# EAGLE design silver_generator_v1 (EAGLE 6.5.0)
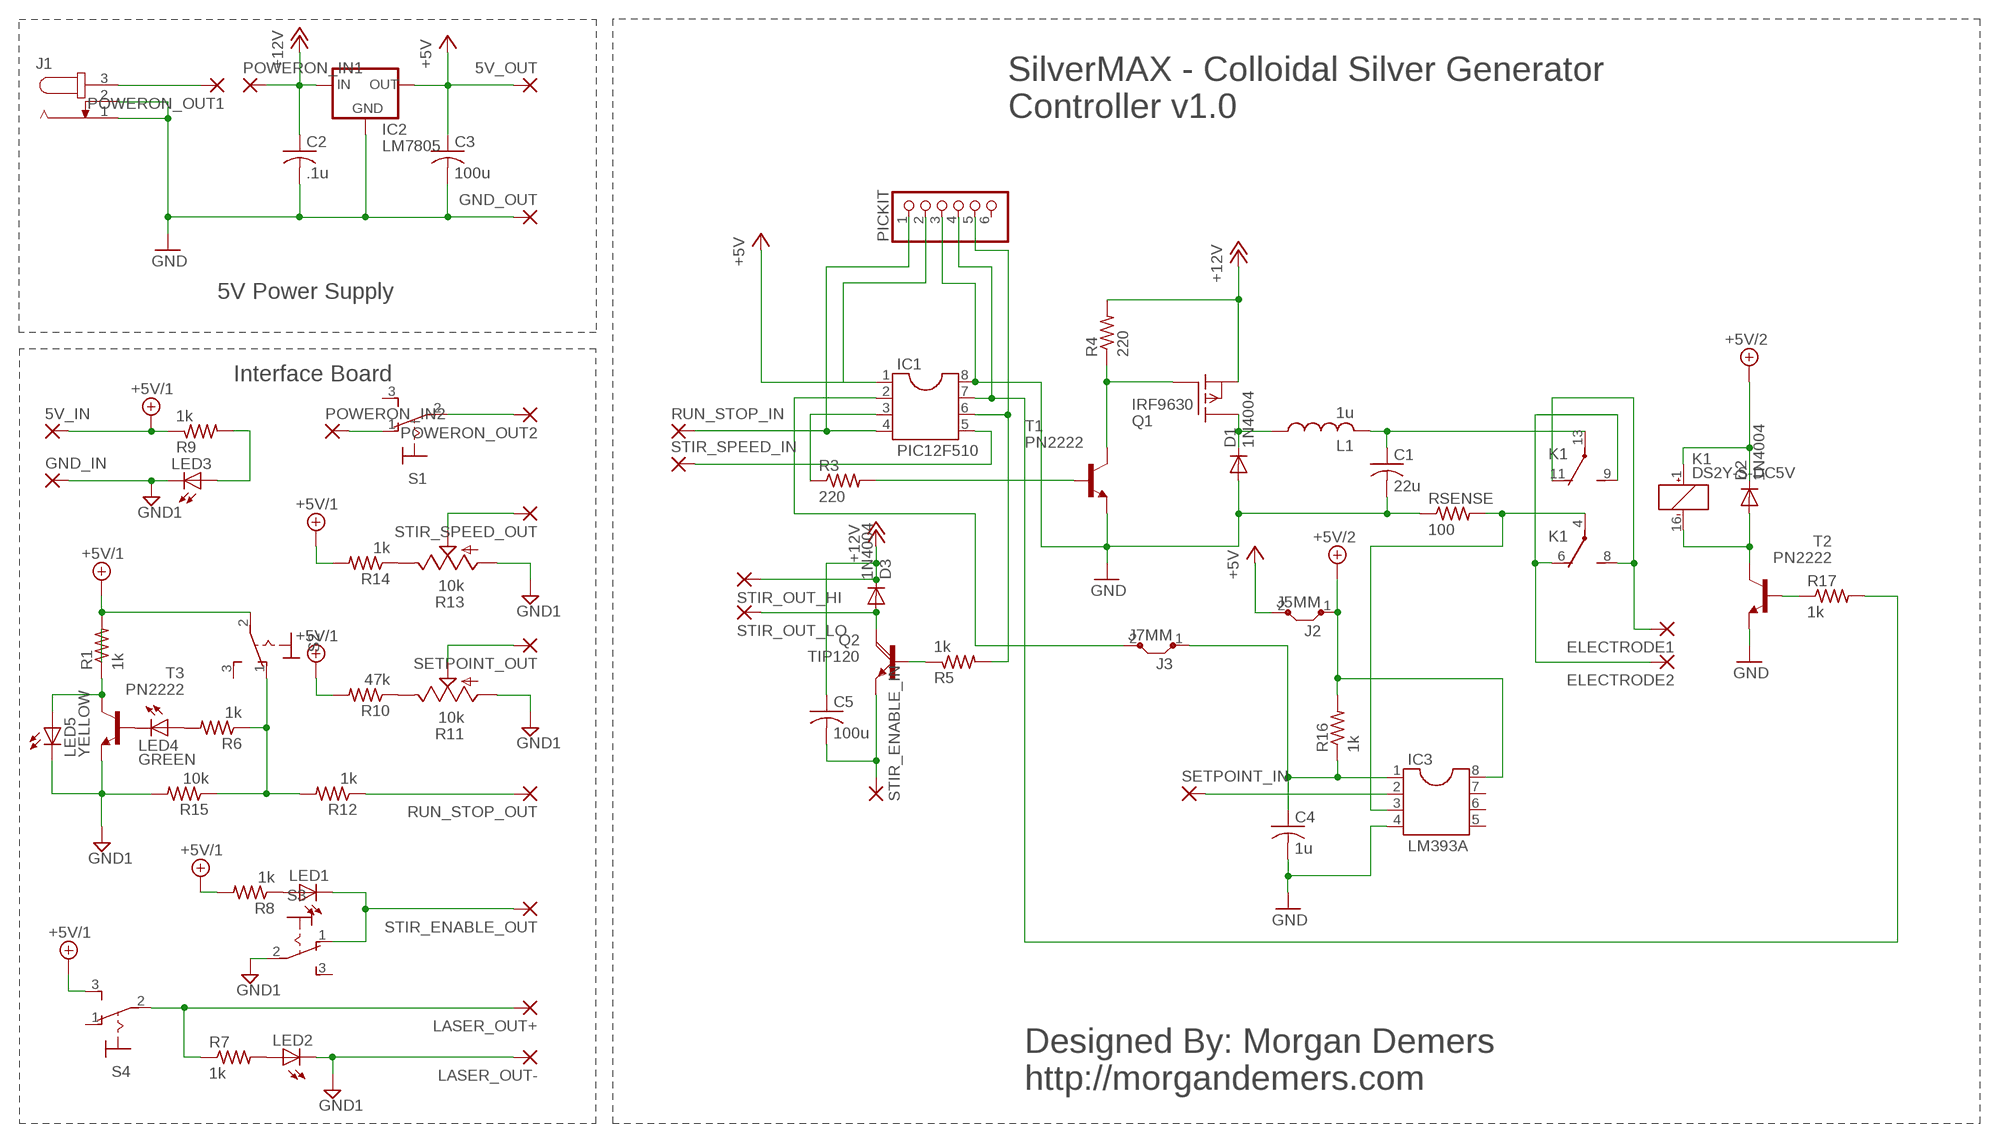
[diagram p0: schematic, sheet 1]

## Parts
5V_IN  1,6/0,9  [1,6/0,9]
5V_OUT  1,6/0,9  [1,6/0,9]
C1  22u  C-US025-050X050  [C025-050X050]
C2  .1u  C-US025-025X050  [C025-025X050]
C3  100u  C-US025-050X050  [C025-050X050]
C4  1u  C-US025-050X050  [C025-050X050]
C5  100u  C-US050-075X075  [C050-075X075]
D1  1N4004  [DO41-10]
D2  1N4004  [DO41-10]
D3  1N4004  [DO41-10]
ELECTRODE1  1,6/0,9  [1,6/0,9]
ELECTRODE2  1,6/0,9  [1,6/0,9]
GND_IN  1,6/0,9  [1,6/0,9]
GND_OUT  1,6/0,9  [1,6/0,9]
IC1  PIC12F510  DIL8S  [SOCKET-08]
IC2  LM7805  78XXL  [78XXL]
IC3  LM393A  DIL8S  [SOCKET-08]
J1  JACK-PLUG1  [SPC4078]
J2  J5MM  [05]
J3  J7MM  [07]
K1  DS2Y-S-DC5V  [DS2Y]
L1  1u  L-US0204/5  [0204/5]
LASER_OUT+  1,6/0,9  [1,6/0,9]
LASER_OUT-  1,6/0,9  [1,6/0,9]
LED1  LED3MM  [LED3MM]
LED2  LED3MM  [LED3MM]
LED3  LED3MM  [LED3MM]
LED4  GREEN  LED3MM  [LED3MM]
LED5  YELLOW  LED3MM  [LED3MM]
PICKIT  PINHD-1X6  [1X06]
POWERON_IN1  1,6/0,9  [1,6/0,9]
POWERON_IN2  1,6/0,9  [1,6/0,9]
POWERON_OUT1  1,6/0,9  [1,6/0,9]
POWERON_OUT2  1,6/0,9  [1,6/0,9]
Q1  IRF9630  IRF9530  [TO220]
Q2  TIP120  [TO220AH]
R1  1k  R-US_0204/5  [0204/5]
R3  220  R-US_0204/7  [0204/7]
R4  220  R-US_0204/5  [0204/5]
R5  1k  R-US_0207/12  [0207/12]
R6  1k  R-US_0204/5  [0204/5]
R7  1k  R-US_0204/5  [0204/5]
R8  1k  R-US_0204/5  [0204/5]
R9  1k  R-US_0204/5  [0204/5]
R10  47k  R-US_0204/5  [0204/5]
R11  10k  TRIM_US-B25P  [B25P]
R12  1k  R-US_0204/5  [0204/5]
R13  10k  TRIM_US-B25P  [B25P]
R14  1k  R-US_0204/5  [0204/5]
R15  10k  R-US_0204/5  [0204/5]
R16  1k  R-US_0204/5  [0204/5]
R17  1k  R-US_0204/7  [0204/7]
RSENSE  100  R-US_0204/5  [0204/5]
RUN_STOP_IN  1,6/0,9  [1,6/0,9]
RUN_STOP_OUT  1,6/0,9  [1,6/0,9]
S1  M9040P  [M9040P]
S2  M9040P  [M9040P]
S3  M9040P  [M9040P]
S4  M9040P  [M9040P]
SETPOINT_IN  1,6/0,9  [1,6/0,9]
SETPOINT_OUT  1,6/0,9  [1,6/0,9]
STIR_ENABLE_IN  1,6/0,9  [1,6/0,9]
STIR_ENABLE_OUT  1,6/0,9  [1,6/0,9]
STIR_OUT_HI  1,6/0,9  [1,6/0,9]
STIR_OUT_LO  1,6/0,9  [1,6/0,9]
STIR_SPEED_IN  1,6/0,9  [1,6/0,9]
STIR_SPEED_OUT  1,6/0,9  [1,6/0,9]
T1  PN2222  -NPN-TO92-EBC  [TO92-EBC]
T2  PN2222  -NPN-TO92-EBC  [TO92-EBC]
T3  PN2222  -NPN-TO92-EBC  [TO92-EBC]

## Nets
+5V: 5V_OUT.1(P) C3.1 IC1.1 IC2.OUT J2.2 PICKIT.2
+5V/1: 5V_IN.1(P) R1.2 R8.2 R9.1 R10.2 R14.2 S2.2(P) S4.3(S)
+5V/2: D2.C IC3.8 J2.1 K1.1(1:+) R16.2
+12V: C2.1 C5.1 D3.C IC2.IN POWERON_IN1.1(P) Q1.3(S) R4.2 STIR_OUT_HI.1(P)
GND: C1.2 C2.2 C3.2 C4.2 D1.A GND_OUT.1(P) IC1.8 IC2.GND IC3.4 J1.1 J1.2 PICKIT.3 RSENSE.1 T1.E T2.E
GND1: GND_IN.1(P) LASER_OUT-.1(P) LED2.K(C) LED3.K(C) LED5.K(C) R11.A R13.A R15.2 S3.2(P) T3.E
N$1: IC1.3 R3.1
N$2: R3.2 T1.B
N$3: LED1.K(C) S3.1(O) STIR_ENABLE_OUT.1(P)
N$4: IC3.2 SETPOINT_IN.1(P)
N$5: Q1.1(G) R4.1 T1.C
N$6: D3.A Q2.C STIR_OUT_LO.1(P)
N$7: C1.1 K1.13(3:P) L1.2
N$8: IC1.6 PICKIT.5 R5.2
N$9: IC1.4 PICKIT.1 RUN_STOP_IN.1(P)
N$10: D1.C L1.1 Q1.2(D)
N$11: POWERON_IN2.1(P) S1.1(O)
N$12: IC3.3 K1.4(2:P) RSENSE.2
N$13: R6.1 R12.2 R15.1 S2.1(O)
N$14: LED2.A R7.2
N$15: ELECTRODE2.1(P) K1.6(2:O) K1.9(3:S)
N$16: LED1.A R8.1
N$17: R13.S STIR_SPEED_OUT.1(P)
N$18: LED3.A R9.2
N$19: IC1.7 PICKIT.4 R17.2
N$20: R10.1 R11.E
N$21: ELECTRODE1.1(P) K1.8(2:S) K1.11(3:O)
N$22: IC1.2 J3.2
N$24: LED5.A R1.1 T3.C
N$25: LED4.K(C) T3.B
N$26: LED4.A R6.2
N$27: LASER_OUT+.1(P) R7.1 S4.2(P)
N$28: C5.2 Q2.E STIR_ENABLE_IN.1(P)
N$29: IC1.5 STIR_SPEED_IN.1(P)
N$30: R13.E R14.1
N$31: Q2.B R5.1
N$32: R12.1 RUN_STOP_OUT.1(P)
N$33: R11.S SETPOINT_OUT.1(P)
N$34: R17.1 T2.B
N$35: D2.A K1.16(1:-) T2.C
N$36: J1.3 POWERON_OUT1.1(P)
N$39: POWERON_OUT2.1(P) S1.2(P)
N$40: C4.1 IC3.1 J3.1 R16.1
Unconnected: IC3.5 IC3.6 IC3.7 PICKIT.6 S1.3(S) S2.3(S) S3.3(S) S4.1(O)

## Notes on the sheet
- SilverMAX - Colloidal Silver Generator
  Controller v1.0
- 5V Power Supply
- Interface Board
- Designed By: Morgan Demers
  http://morgandemers.com

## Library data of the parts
5V_IN 5V_OUT ELECTRODE1 ELECTRODE2 GND_IN GND_OUT LASER_OUT+ LASER_OUT- POWERON_IN1 POWERON_IN2 POWERON_OUT1 POWERON_OUT2 RUN_STOP_IN RUN_STOP_OUT SETPOINT_IN SETPOINT_OUT STIR_ENABLE_IN STIR_ENABLE_OUT STIR_OUT_HI STIR_OUT_LO STIR_SPEED_IN STIR_SPEED_OUT = wirepad:1,6/0,9: THROUGH-HOLE PAD
C1-C5 = resistor:C-US: CAPACITOR, American symbol
D1-D3 = diode:1N4004: DIODE
IC1 IC3 = ic-package:DIL8: Dual In Line / Socket
IC2 = v-reg:78XXL: VOLTAGE REGULATOR
J1 = con-jack:JACK-PLUG: DC POWER JACK Power Jack, DC, Right Angle, Through Hole, Rated 5A at 16VDC, PC Terminals Distributor: Farnell (www.Farnell.de) Drawing: 84N1161.pdf / 84N1162.pdf Manufacturer: SPC Technology (www.spctechnology.com) Type: SPC4077 / SPC 4078; OC_FARNELL: unknown; OC_NEWARK: unknown
J2 J3 = jumper:J: Bridge
K1 = relay:DS2Y-S-DC*: MINIATURE RELAY NAiS Source: http://www.mew-europe.com/.. en_ds_61005_0023.pdf; MPN: DS2Y-S-DC5V; OC_FARNELL: unknown; OC_NEWARK: 13P3268
L1 = resistor:L-US: INDUCTOR, American symbol
LED1-LED5 = led:LED: LED
PICKIT = pinhead:PINHD-1X6: PIN HEADER
Q1 = transistor-fet:IRF9530: P-Channel Enhancement MOSFET (HEXFET); -100V; -12A; 0,3Ohm
Q2 = transistor-power:TIP120: NPN DARLINGTON TRANSISTOR
R1 R3-R10 R12 R14-R17 RSENSE = resistor:R-US_: RESISTOR, American symbol
R11 R13 = pot:TRIM_US-: POTENTIOMETER
S1-S4 = switch:M9040P: TOGGLE SWITCH Marquardt
T1-T3 = transistor:*-NPN-: NPN Transistror BF959 corrected 2008.03.06

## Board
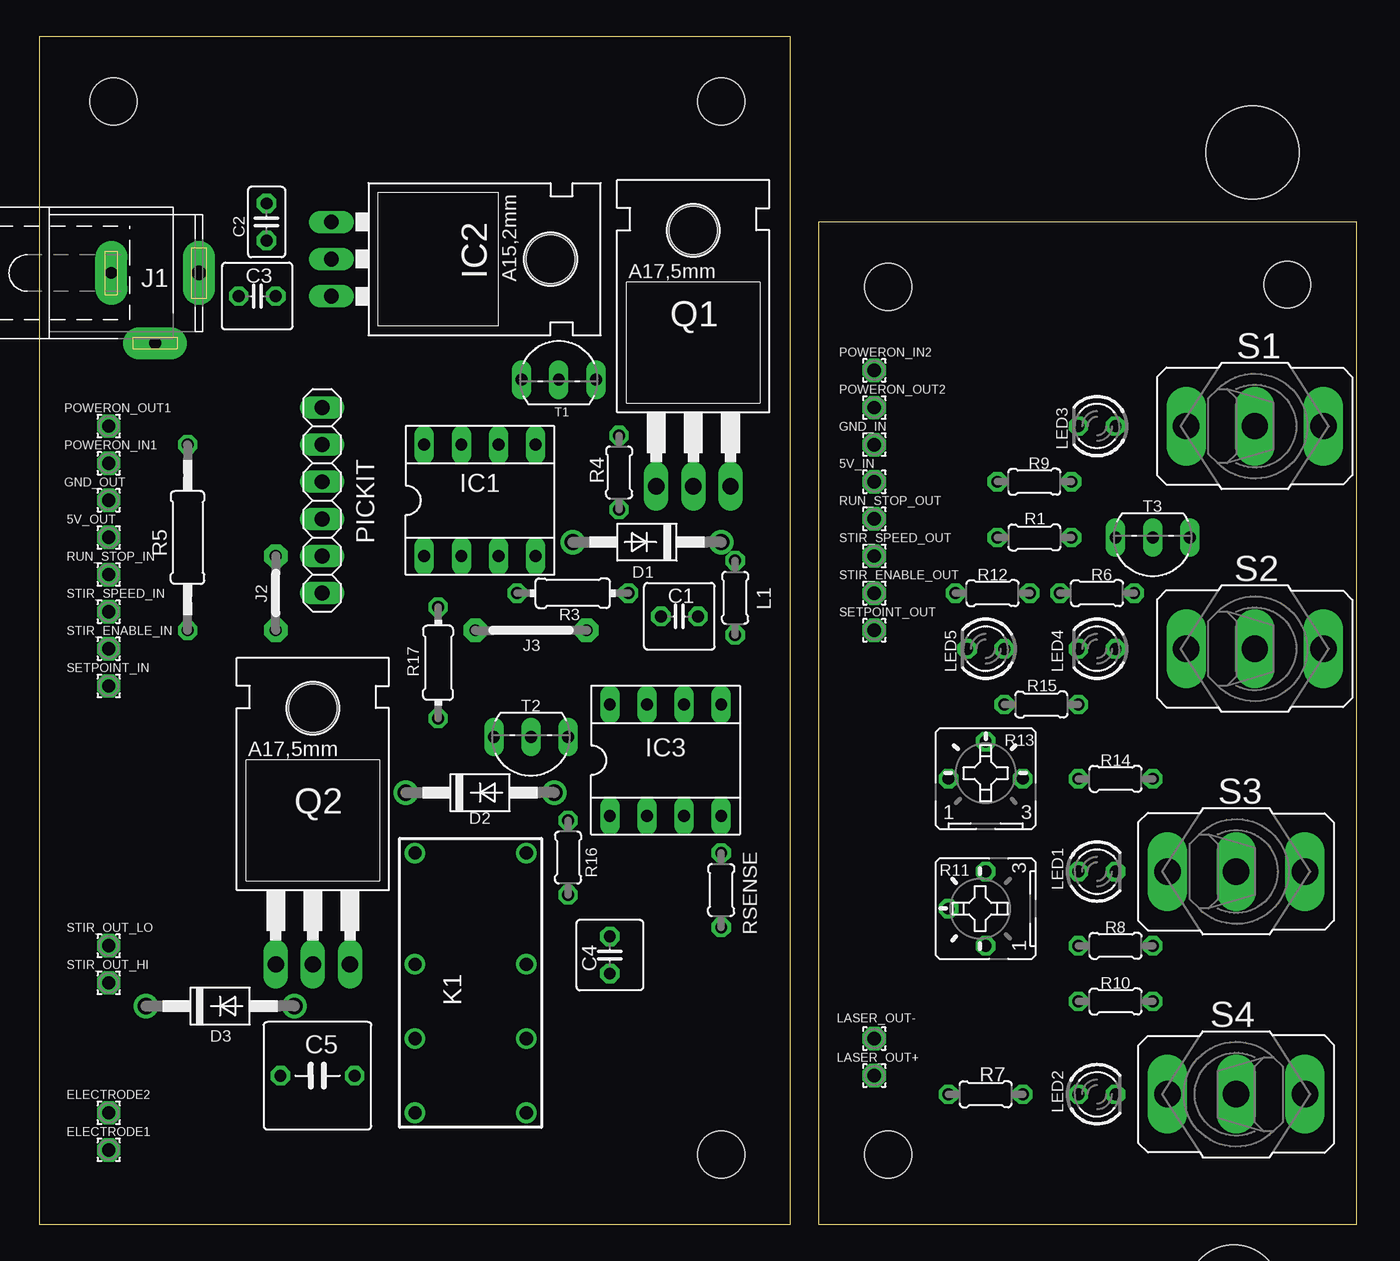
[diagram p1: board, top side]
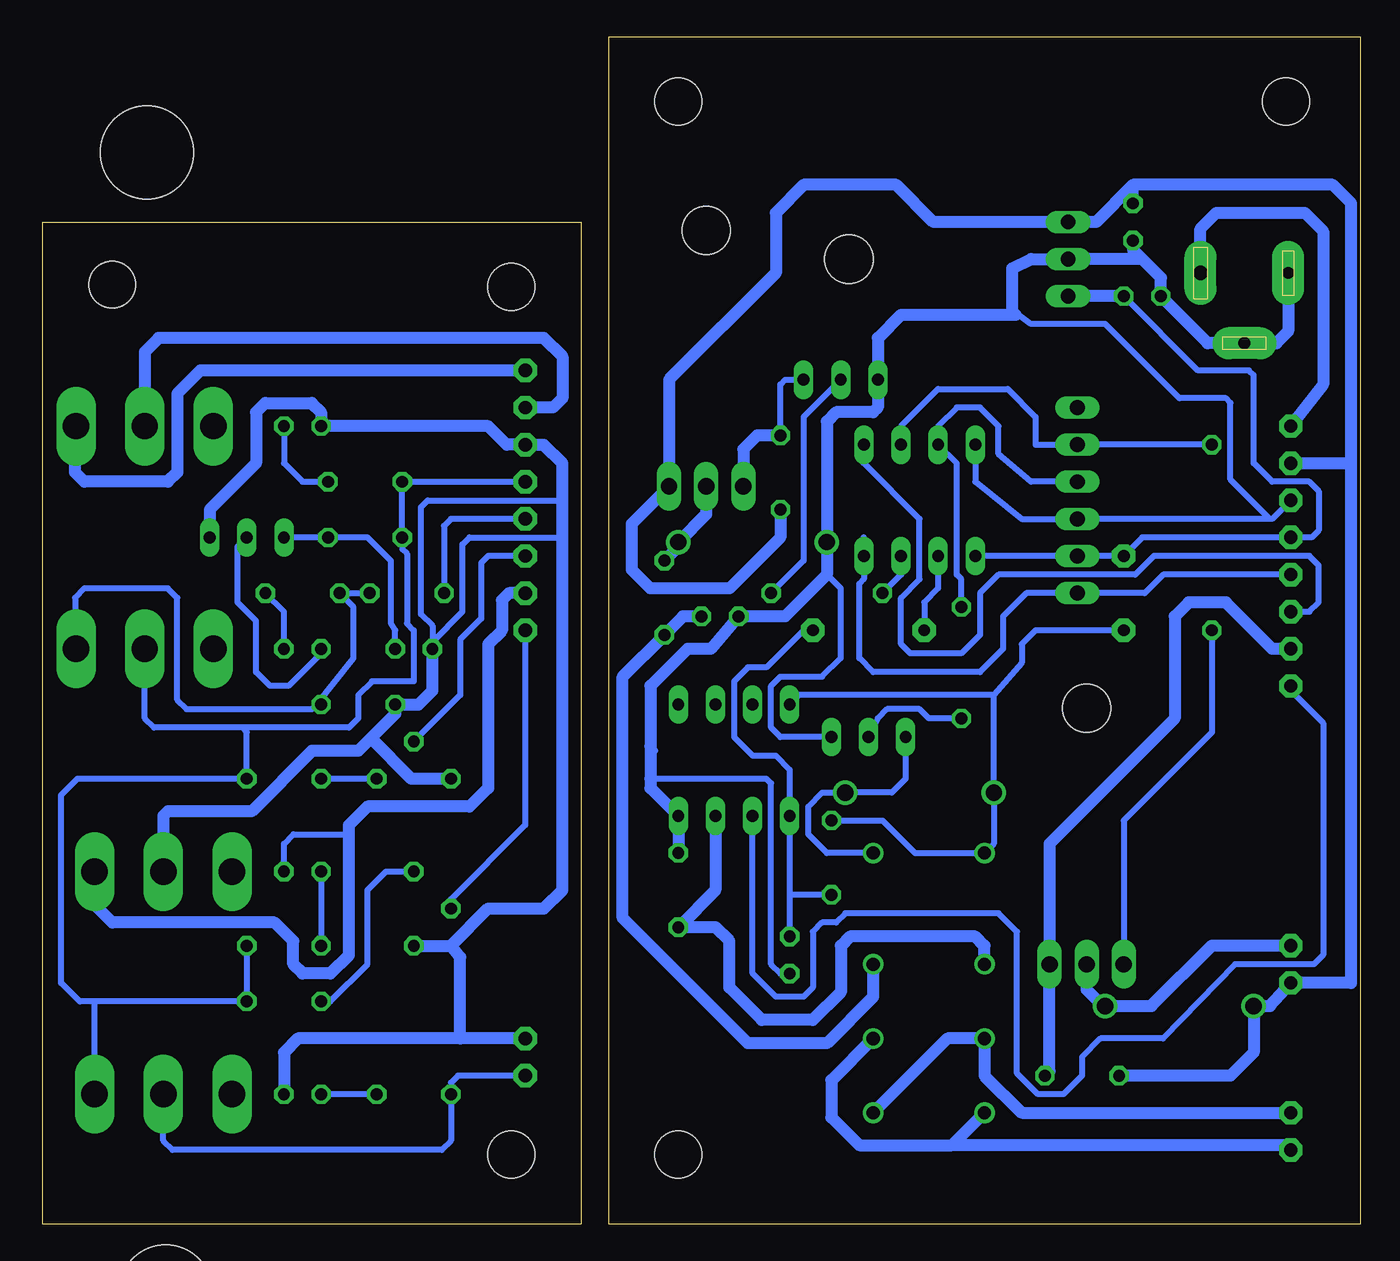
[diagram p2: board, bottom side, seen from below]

Size 90.17 x 81.27 mm. Coordinates in mm from the lower left corner, seen from the top.
Outline: 0,0 51.42,0 51.42,81.27 0,81.27 0,0
Outline: 53.34,68.58 53.34,0 90.17,0 90.17,68.58 53.34,68.58
Copper layers (1*16): Top 0.035mm / dielectric 1.5mm / Bottom 0.035mm
Design rules "default": minimum track width 10mil, minimum drill 24mil, track to track 8mil, track to pad 8mil, pad to pad 8mil, via to via 8mil, smd to smd 8mil, copper to edge 40mil, drill to drill 8mil, minimum pad ring 10mil, minimum via ring 8mil, stop-mask expansion 4mil, vias tented up to drill 0mil, thermal gap 10mil
Holes 3.2 mm at 5.08,76.83 46.67,76.83 46.67,4.76 58.1,4.76 85.41,64.29 58.1,64.14
Holes 6.35 mm at 83.03,73.34 81.76,-4.6

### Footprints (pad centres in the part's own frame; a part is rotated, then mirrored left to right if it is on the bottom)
1,6/0,9 = drill 0.914 pad 1.6 octagon: 1 0,0
C025-050X050 = drill 0.813 octagon: 1 -1.27,0; 2 1.27,0
C025-025X050 = drill 0.813 octagon: 1 -1.27,0; 2 1.27,0
C050-075X075 = drill 0.813 octagon: 1 -2.54,0; 2 2.54,0
DO41-10 = drill 1.118: A 5.08,0; C -5.08,0
SOCKET-08 = drill 0.813 long: 1 -3.81,-3.81; 2 -1.27,-3.81; 3 1.27,-3.81; 4 3.81,-3.81; 5 3.81,3.81; 6 1.27,3.81; 7 -1.27,3.81; 8 -3.81,3.81
78XXL = drill 1.016 long: GND 0,-3.81; IN -2.54,-3.81; OUT 2.54,-3.81 | hole 3.302: 0,11.176
SPC4078 = drill 0.8 pad 2.184 long: 1 -3,0; 2 0,-4.8 | drill 1 pad 2.184 long: 3 3,0
05 = drill 0.813 pad 1.6 octagon: 1 -2.54,0; 2 2.54,0
07 = drill 0.813 pad 1.6 octagon: 1 -3.81,0; 2 3.81,0
DS2Y = drill 0.9: 1 -8.89,-3.81; 4 -1.27,-3.81; 6 3.81,-3.81; 8 8.89,-3.81; 9 8.89,3.81; 11 3.81,3.81; 13 -1.27,3.81; 16 -8.89,3.81
0204/5 = drill 0.813 octagon: 1 -2.54,0; 2 2.54,0
LED3MM = drill 0.813 octagon: A -1.27,0; K 1.27,0
1X06 = drill 1.016 long: 1 -6.35,0; 2 -3.81,0; 3 -1.27,0; 4 1.27,0; 5 3.81,0; 6 6.35,0
TO220 = drill 1.118 long: 1 -2.54,-6.35; 2 0,-6.35; 3 2.54,-6.35 | hole 3.302: 0,11.176
TO220AH = drill 1.118 long: B -2.54,-6.35; C 0,-6.35; E 2.54,-6.35 | hole 3.302: 0,11.176
0204/7 = drill 0.813 octagon: 1 -3.81,0; 2 3.81,0
0207/12 = drill 0.813 octagon: 1 -6.35,0; 2 6.35,0
B25P = drill 0.813 octagon: A -2.54,0; E 2.54,0; S 0,2.54
M9040P = drill 1.803 long: 1 0,4.699; 2 0,0; 3 0,-4.699
TO92-EBC = drill 0.813 long: B 0,-1.27; C 2.54,-1.27; E -2.54,-1.27

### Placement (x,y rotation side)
5V_IN  57.15,50.8 0 top
5V_OUT  4.76,46.99 0 top
C1  43.81,41.59 180 top
C2  15.56,68.58 270 top
C3  14.92,63.5 180 top
C4  39.05,18.41 270 top
C5  19.05,10.16 0 top
D1  41.59,46.67 180 top
D2  30.16,29.53 0 top
D3  12.38,14.92 0 top
ELECTRODE1  4.76,5.08 0 top
ELECTRODE2  4.76,7.62 0 top
GND_IN  57.15,53.34 0 top
GND_OUT  4.76,49.53 0 top
IC1  30.16,49.53 0 top
IC2  23.81,66.04 270 top
IC3  42.86,31.75 0 top
J1  7.94,65.09 0 top
J2  16.19,43.18 90 top
J3  33.66,40.64 180 top
K1  29.53,16.51 270 top
L1  47.62,42.86 270 top
LASER_OUT+  57.15,10.16 0 top
LASER_OUT-  57.15,12.7 0 top
LED1  72.39,24.13 0 top
LED2  72.39,8.89 0 top
LED3  72.39,54.61 180 top
LED4  72.39,39.37 180 top
LED5  64.77,39.37 180 top
PICKIT  19.37,49.53 90 top
POWERON_IN1  4.76,52.07 0 top
POWERON_IN2  57.15,58.42 0 top
POWERON_OUT1  4.76,54.61 0 top
POWERON_OUT2  57.15,55.88 0 top
Q1  44.77,56.83 0 top
Q2  18.73,24.13 0 top
R1  68.1,46.99 180 top
R3  36.51,43.18 0 top
R4  39.69,51.44 270 top
R5  10.16,46.99 90 top
R6  72.39,43.18 0 top
R7  64.77,8.89 0 top
R8  73.66,19.05 0 top
R9  68.1,50.8 0 top
R10  73.66,15.24 0 top
R11  64.77,21.59 90 top
R12  65.25,43.18 0 top
R13  64.77,30.48 0 top
R14  73.66,30.48 0 top
R15  68.58,35.56 180 top
R16  36.2,25.08 90 top
R17  27.3,38.42 90 top
RSENSE  46.67,22.86 270 top
RUN_STOP_IN  4.76,44.45 0 top
RUN_STOP_OUT  57.15,48.26 0 top
S1  83.19,54.61 270 top
S2  83.19,39.37 270 top
S3  81.92,24.13 270 top
S4  81.92,8.89 90 top
SETPOINT_IN  4.76,36.83 0 top
SETPOINT_OUT  57.15,40.64 0 top
STIR_ENABLE_IN  4.76,39.37 0 top
STIR_ENABLE_OUT  57.15,43.18 0 top
STIR_OUT_HI  4.76,16.51 0 top
STIR_OUT_LO  4.76,19.05 0 top
STIR_SPEED_IN  4.76,41.91 0 top
STIR_SPEED_OUT  57.15,45.72 0 top
T1  35.56,59.05 0 top
T2  33.66,32.07 180 top
T3  76.2,45.72 180 top

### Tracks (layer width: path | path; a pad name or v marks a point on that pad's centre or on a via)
+5V
  Bottom 0.406: IC1.1 PICKIT.2 J2.2 14.92,46.99 5V_OUT.1 3.33,46.99 2.86,47.47 2.86,50.16 3.49,50.8 6.03,50.8 7.3,52.07 7.3,58.1 7.62,58.42 11.11,58.42 C3.1
  Bottom 0.813: C3.1 IC2.OUT
+5V/1
  Bottom 0.406: 5V_IN.1 R9.1 R1.2 65.56,46.2 65.25,45.88 65.25,41.12 64.77,40.64 64.77,37.15 67.63,37.15 68.58,36.2 68.58,34.61 69.22,33.97 76.52,33.97 | 76.52,33.97 82.55,33.97 83.19,34.61 S2.2 | R10.2 76.83,15.24 | 76.83,15.24 86.68,15.24 | R8.2 76.2,15.88 76.83,15.24 | 76.52,33.97 76.2,33.66 R14.2 87.79,30.48 88.9,29.37 88.9,16.51 87.63,15.24 86.68,15.24 | S4.3 86.61,15.18 86.68,15.24
+5V/2
  Bottom 0.406: 25.08,36.2 23.18,38.42 23.18,39.69 22.23,40.64 J2.1 | 25.08,36.2 38.42,36.2 IC3.8 | 25.08,36.2 D2.C 25.08,26.04 K1.1 30.48,25.4 32.7,27.62 R16.2
+12V
  Bottom 0.813: 15.56,71.12 1.91,71.12 0.64,69.85 0.64,52.07 | 15.56,71.12 18.1,68.58 IC2.IN 29.21,68.58 31.75,71.12 38.1,71.12 40.01,69.22 40.01,65.09 47.31,57.78 Q1.3 49.85,47.94 49.85,44.77 48.58,43.5 43.18,43.5 39.69,46.99 R4.2 | C2.1 15.56,71.12 | 0.64,52.07 0.64,16.51 STIR_OUT_HI.1 6.19,14.92 D3.C 7.3,11.75 8.89,10.16 C5.1 | POWERON_IN1.1 0.64,52.07
GND
  Bottom 0.406: IC1.8 26.35,50.8 23.18,48.26 PICKIT.3 | GND_OUT.1 6.03,48.26 6.19,48.26 | 6.19,48.26 PICKIT.3 | PICKIT.3 18.73,48.26 | 23.51,62.32 22.54,61.59 17.46,61.59 12.38,56.52 9.21,56.52 8.89,56.2 8.89,50.96 6.19,48.26 | 23.51,62.32 23.81,62.55 | 23.6,62.23 23.51,62.32 | C4.2 39.69,17.14 40.32,17.78 40.32,30.16 40.64,30.48 48.58,30.48 | 48.26,32.38 48.58,32.7 | T2.E 39.69,33.34 40.32,33.97 40.32,36.83 39.69,37.47 36.83,37.47 35.56,38.73 35.56,43.5 36.51,44.45
  Bottom 0.813: 14.92,66.04 13.65,64.77 C3.2 10.44,60.29 J1.2 5.75,60.29 4.94,61.1 J1.1 | 14.92,66.04 IC2.GND 22.54,66.04 23.81,65.41 23.81,62.55 | C2.2 15.56,66.67 14.92,66.04 | 23.6,62.23 31.43,62.23 33.02,60.64 T1.E 33.02,55.88 33.34,55.56 35.88,55.56 36.51,54.93 D1.A 36.51,44.45 39.37,41.59 C1.2 44.45,39.37 46.04,39.37 48.58,36.83 48.58,32.7 48.58,30.48 48.58,29.84 IC3.4 RSENSE.1
GND1
  Bottom 0.406: 54.61,49.53 63.82,49.53 64.29,49.05 64.29,41.75 63.5,40.96 63.5,39.85 | 63.5,39.85 61.44,41.91 61.44,46.51 60.96,46.99 54.93,46.99 54.77,46.83 | 63.5,39.85 LED5.K
  Bottom 0.813: R11.A 62.23,19.05 | 62.23,19.05 61.59,18.26 61.59,12.7 | 62.23,19.05 59.69,21.59 55.88,21.59 54.61,22.86 54.61,49.53 54.61,52.07 55.88,53.34 GND_IN.1 58.42,53.34 59.69,54.61 LED3.K 71.12,55.56 71.75,56.2 74.93,56.2 75.56,55.56 75.56,52.07 78.74,48.9 T3.E | LASER_OUT-.1 61.59,12.7 | 61.59,12.7 72.71,12.7 73.66,11.75 LED2.K | 67.71,33.26 66.04,34.92 R15.2 64.45,35.56 63.5,36.51 LED5.K | 67.71,33.26 68.58,32.38 71.75,32.38 75.88,28.26 81.6,28.26 81.92,27.94 S3.2 | R13.A 64.93,30.48 67.71,33.26
N$1
  Bottom 0.406: IC1.3 31.43,44.45 R3.1
N$2
  Bottom 0.406: R3.2 38.1,45.4 38.1,55.24 T1.B
N$3
  Bottom 0.406: LED1.K 73.66,26.04 73.03,26.67 69.22,26.67
  Bottom 0.813: S3.1 86.68,24.07 86.68,21.91 85.41,20.64 74.3,20.64 73.03,19.37 73.03,17.78 72.39,17.14 70.48,17.14 69.22,18.41 69.22,26.67 69.22,27.3 67.94,28.57 60.96,28.57 59.69,29.84 59.69,39.69 58.74,40.64 58.74,42.7 58.26,43.18 STIR_ENABLE_OUT.1
N$4
  Bottom 0.406: IC3.2 41.59,17.14 40.01,15.56 38.1,15.56 37.47,16.19 37.47,20 36.83,20.64 35.88,20.64 35.24,21.27 24.77,21.27 23.5,20 23.5,10.32 22.07,8.89 20.32,8.89 19.05,10.16 19.05,11.43 17.78,12.7 13.49,12.7 8.57,17.78 3.17,17.78 2.54,18.41 2.54,34.29 4.76,36.51 SETPOINT_IN.1
N$5
  Bottom 0.406: R4.1 39.69,57.47 39.37,57.78 T1.C
  Bottom 0.813: R4.1 41.27,53.98 42.23,53.02 Q1.1
N$6
  Bottom 0.813: STIR_OUT_LO.1 10.16,19.05 14.29,14.92 D3.A 17.62,14.92 18.73,16.03 Q2.C
N$7
  Bottom 0.813: C1.1 46.35,41.59 L1.2 50.48,37.47 50.48,20.95 41.91,12.38 36.51,12.38 33.34,15.56 K1.13
N$8
  Bottom 0.406: IC1.6 31.43,54.61 28.89,57.15 24.13,57.15 22.23,55.24 22.23,53.34 PICKIT.5 | 19.68,53.66 PICKIT.5 | R5.2 PICKIT.5
N$9
  Bottom 0.406: 33.97,46.99 IC1.4 33.97,44.13 34.29,43.81 34.29,38.73 33.34,37.78 26.04,37.78 24.45,39.37 24.45,41.59 22.86,43.18 PICKIT.1 14.76,43.18 13.49,44.45 RUN_STOP_IN.1
N$10
  Bottom 0.813: L1.1 46.67,46.35 D1.C 44.77,48.58 Q1.2
N$11
  Bottom 0.813: POWERON_IN2.1 79.38,58.42 80.96,56.83 80.96,51.44 81.6,50.8 87.31,50.8 87.95,51.44 87.95,54.55 S1.1
N$12
  Bottom 0.813: IC3.3 44.13,22.86 RSENSE.2 44.13,20.32 43.18,19.37 43.18,16.19 40.96,13.97 37.47,13.97 35.56,15.88 35.56,19.05 34.92,19.68 26.35,19.68 25.72,19.05 K1.4
N$13
  Bottom 0.406: 71.44,35.56 68.9,38.73 68.9,42.23 R6.1 R12.2 | R15.1 71.44,35.56 | 71.44,35.56 71.75,35.24 80.33,35.24 80.96,35.88 80.96,42.86 81.6,43.5 87.31,43.5 87.95,42.86 87.95,39.43 S2.1
N$14
  Bottom 0.406: R7.2 LED2.A
N$15
  Bottom 0.813: K1.9 28.26,12.7 K1.6 25.72,10.16 23.18,7.62 ELECTRODE2.1
N$16
  Bottom 0.406: LED1.A R8.1
N$17
  Bottom 0.406: STIR_SPEED_OUT.1 59.69,45.72 60.17,45.24 60.17,41.43 61.59,40.01 61.59,36.2 R13.S
N$18
  Bottom 0.406: LED3.A 73.66,52.07 72.39,50.8 R9.2
N$19
  Bottom 0.406: PICKIT.4 22.54,50.8 24.77,52.7 24.77,54.61 26.04,55.88 27.62,55.88 28.89,54.61 IC1.7 27.62,52.07 27.62,44.45 27.3,44.13 R17.2
N$20
  Bottom 0.406: R10.1 70.48,15.24 67.94,17.78 67.94,22.86 66.67,24.13 R11.E
N$21
  Bottom 0.813: K1.11 36.2,9.84 36.2,7.3 34.29,5.4 27.94,5.4 | K1.8 27.94,5.4 | ELECTRODE1.1 5.08,5.4 27.94,5.4
N$22
  Bottom 0.406: IC1.2 28.89,43.5 29.84,42.55 J3.2
N$24
  Bottom 0.406: LED5.A 66.04,40.64 66.36,41.12 66.36,45.4 67.94,46.99 R1.1 T3.C
N$25
  Bottom 0.406: LED4.K 71.12,39.05 73.34,36.83 74.61,36.83 75.56,37.78 75.56,41.27 76.83,42.55 76.83,46.35 T3.B
N$26
  Bottom 0.406: LED4.A 73.66,41.91 R6.2
N$27
  Bottom 0.406: LASER_OUT+.1 61.75,10.16 62.23,9.68 R7.1 62.23,5.71 62.87,5.08 81.28,5.08 81.92,5.71 S4.2
N$28
  Bottom 0.813: STIR_ENABLE_IN.1 6.03,39.37 9.21,42.55 11.75,42.55 12.7,41.59 12.7,34.61 21.27,26.04 Q2.E 21.27,10.48 C5.2
N$29
  Bottom 0.406: STIR_SPEED_IN.1 3.49,41.91 2.86,42.55 2.86,45.09 3.49,45.72 14.13,45.72 15.4,44.45 24.77,44.45 26.04,43.18 26.04,40.32 27.3,39.05 30.8,39.05 31.43,39.69 31.43,42.86 30.16,44.13 30.16,48.26 33.97,52.07 IC1.5
N$30
  Bottom 0.406: R13.E R14.1
N$31
  Bottom 0.406: R5.1 10.16,33.66 16.19,27.62 Q2.B
N$32
  Bottom 0.406: RUN_STOP_OUT.1 62.23,48.26 62.71,47.78 R12.1
N$33
  Bottom 0.406: SETPOINT_OUT.1 57.15,27.3 62.23,22.23 R11.S
N$34
  Bottom 0.406: R17.1 29.53,34.61 30.16,35.24 32.38,35.24 33.02,34.61 T2.B
N$35
  Bottom 0.406: K1.16 36.51,25.4 37.78,26.67 37.78,28.57 36.83,29.53 D2.A 32.07,29.53 31.11,30.48 T2.C
N$36
  Bottom 0.813: J1.3 10.94,68.12 9.84,69.22 3.81,69.22 2.54,67.94 2.54,57.47 POWERON_OUT1.1
N$39
  Bottom 0.813: S1.2 83.19,59.69 82.23,60.64 55.88,60.64 54.61,59.37 54.61,56.52 55.24,55.88 POWERON_OUT2.1
N$40
  Bottom 0.406: 39.05,22.54 IC3.1 39.05,31.11 40.01,32.07 41.59,32.07 42.86,33.34 42.86,37.15 41.91,38.1 40.64,38.1 38.1,40.64 J3.1 | 39.05,22.54 C4.1 | R16.1 39.05,22.54

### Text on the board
200bmp: SilverMAX - Colloidal Silver Generator / Controller Board v1.0 | SilverMAX - C.S. Generator / Interface Board v1.0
